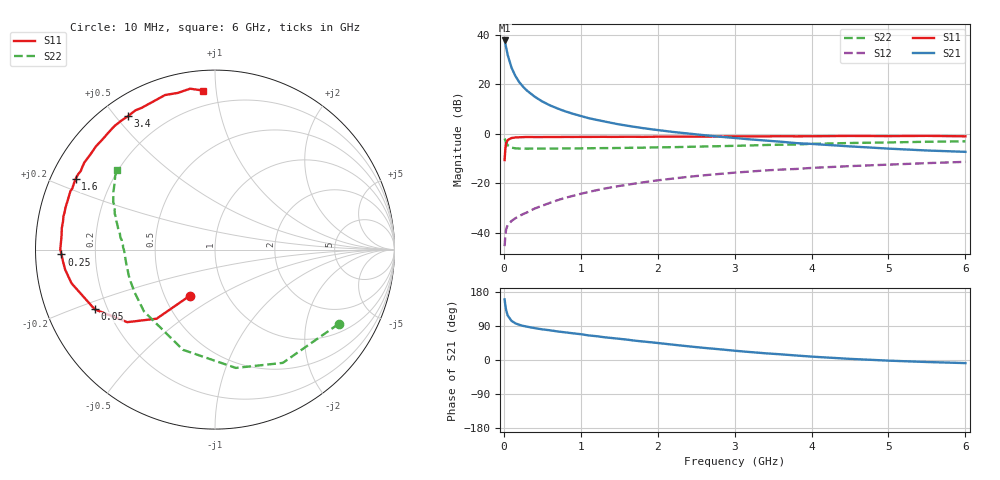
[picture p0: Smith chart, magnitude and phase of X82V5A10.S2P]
! SIEMENS Small Signal Semiconductors
! BFP136W
! Si NPN RF Bipolar Junction Transistor in SOT343
! VCE = 2.5 V  IC = 100 mA
! Common Emitter S-Parameters:  September  1994
# GHz  S  MA  R  50
!  f  S11  S21  S12  S22
! GHz  MAG  ANG  MAG  ANG  MAG  ANG  MAG  ANG
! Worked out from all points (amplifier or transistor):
!   40 points, 10 MHz to 6 GHz, reference 50 ohm
!   highest |S21| = 37.8 dB at 10 MHz (marker M1)
!   |S21| within 3 dB of that: start of sweep to 30.83 MHz
!   unconditionally stable (mu >= 1): 489.6 MHz to 2.893 GHz
!   at 200 MHz: K = 0.70, MSG = 27.1 dB, |S12| = -33.3 dB
!   at 1.5 GHz: K = 1.10, MAG = 10.5 dB, |S12| = -21.1 dB
!   at 6 GHz: K = 0.98, MSG = 2.0 dB, |S12| = -11.4 dB
!   S11 on the Smith chart (normalised r, x): 10 MHz: 0.67, -0.38; 50 MHz: 0.15, -0.23; 250 MHz: 0.08, -0.02; 1.6 GHz: 0.07, +0.24; 3.4 GHz: 0.08, +0.54; 6 GHz: 0.11, +0.92
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0.01  0.2937 -118.7  77.67 159.9  0.0053 68.9  0.8039 -31.0
0.02  0.5041 -130.2  66.34 143.3  0.0089 57.1  0.7356 -59.1
0.03  0.6342 -140.4  55.77 131.5  0.0117 48.3  0.6695 -80.0
0.05  0.7483 -153.6  39.59 117.5  0.0142 38.2  0.5861 -107.7
0.1  0.8212 -166.8  21.81 103.2  0.0172 36.8  0.5245 -139.0
0.15  0.8422 -172.4  14.82 96.8  0.0195 39.7  0.5074 -152.0
0.2  0.8497 -175.6  11.13 92.9  0.0216 42.1  0.5029 -159.0
0.25  0.8558 -178.2  8.977 90.1  0.0237 45.7  0.5019 -163.4
0.3  0.8622 179.9  7.51 88.0  0.0255 48.3  0.4999 -166.4
0.4  0.8587 176.6  5.656 84.1  0.0306 52.8  0.5006 -170.5
0.5  0.8589 174.0  4.508 80.9  0.035 55.3  0.5012 -173.1
0.6  0.8619 172.1  3.764 78.4  0.04 57.9  0.5023 -175.0
0.7  0.8611 169.5  3.246 75.3  0.0453 59.7  0.5032 -176.3
0.9  0.8634 166.1  2.541 70.4  0.0554 60.7  0.5054 -178.8
1.1  0.8651 161.8  2.078 64.9  0.0663 61.4  0.5095 179.5
1.6  0.8709 153.1  1.462 53.8  0.0926 59.8  0.5195 175.5
2.2  0.8734 142.8  1.09 40.4  0.124 55.4  0.536 170.9
3.2  0.8881 126.0  0.771 21.0  0.172 46.0  0.5802 162.1
3.4  0.8877 123.0  0.73 17.7  0.1813 43.8  0.5932 160.3
4.5  0.905 107.9  0.556 3.0  0.2216 33.4  0.6507 150.5
5.5  0.9072 98.8  0.459 -5.3  0.2546 25.5  0.6896 143.8
6  0.8889 94.4  0.431 -8.2  0.2704 21.2  0.7043 140.9
